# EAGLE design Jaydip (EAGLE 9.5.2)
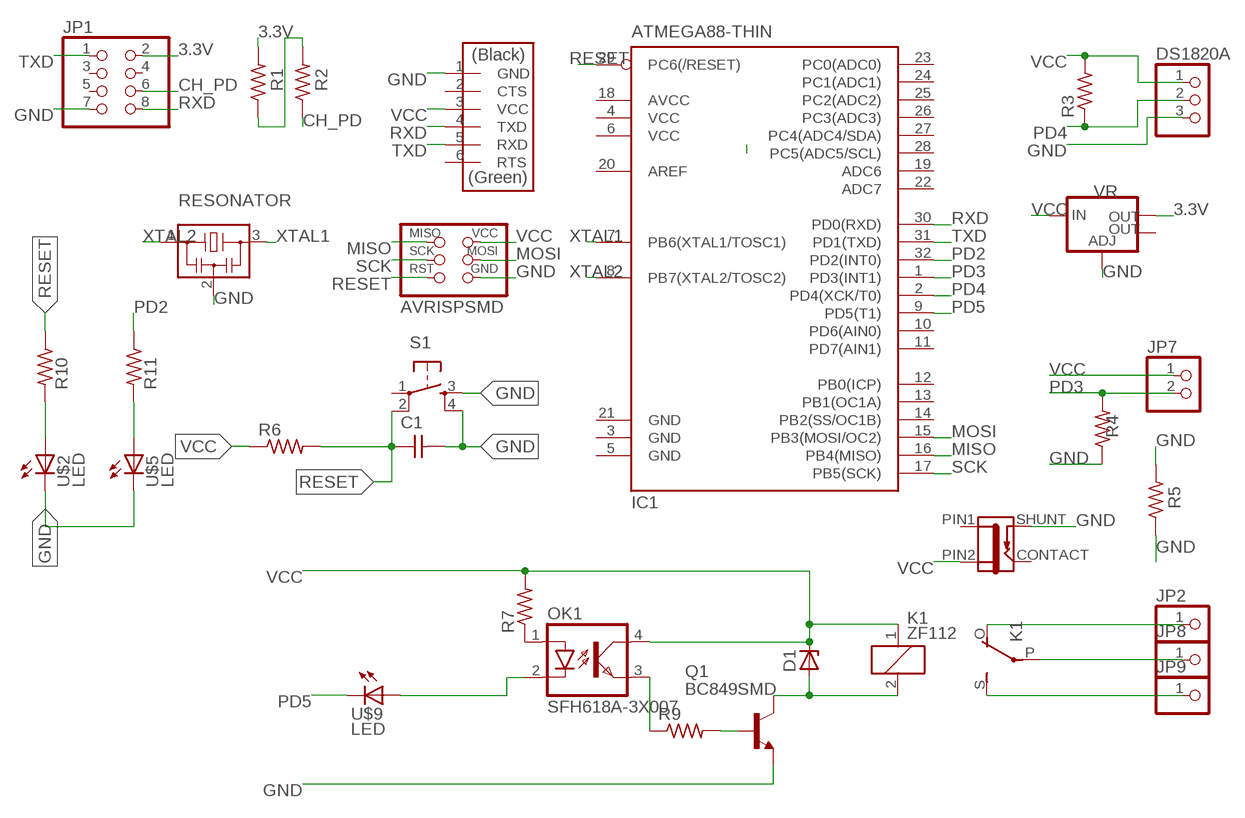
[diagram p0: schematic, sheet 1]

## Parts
C1  CAP-UNPOLARIZED  [C1206]
D1  ZENER_DIODESOD123  [SOD123]
DS1820A  PINHD-1X3  [1X03]
IC1  ATMEGA88-THIN  [TQFP32-08THIN]
J1  JACK-2.1MM  [PJ-002AH-SMT]
JP1  PINHD-2X04_2.54-SMD  [2X04SMD]
JP2  PINHD-1X01_2.00  [1X01M]
JP7  PINHD-1X02_2.54  [1X02]
JP8  PINHD-1X01_2.00  [1X01M]
JP9  PINHD-1X01_2.00  [1X01M]
K1  ZF112  [ZF112]
OK1  SFH618A-3X007  [SMD4-7]
Q1  BC849SMD  [SOT23-BEC]
R1  RES-US1206FAB  [R1206FAB]
R2  RES-US1206FAB  [R1206FAB]
R3  RES-US1206FAB  [R1206FAB]
R4  RES-US1206FAB  [R1206FAB]
R5  RES-US1206FAB  [R1206FAB]
R6  RES-US1206  [R1206]
R7  RES-US1206  [R1206]
R9  RES-US1206  [R1206]
R10  RES-US1206  [R1206]
R11  RES-US1206  [R1206]
S1  6MM_SWITCH6MM_SWITCH  [6MM_SWITCH]
U$1  AVRISPSMD  [2X03SMD]
U$2  LED  [LED1206]
U$3  RESONATOR  [EFOBM]
U$5  LED  [LED1206]
U$7  FTDI-SMD-HEADER  [1X06SMD]
U$9  LED  [LED1206]
VR  V_REG_LM1117SOT223  [SOT223]

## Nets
3.3V: JP1.2 R1.2 VR.2(OUT)
CH_PD: JP1.6 R2.1
GND: C1.2 DS1820A.3 J1.SHUNT JP1.7 Q1.E R4.1 R5.1 R5.2 S1.3(S) S1.4(S1) U$1.6(GND) U$2.2(C) U$3.2 U$5.2(C) U$7.1(GND) VR.1(ADJ)
MISO: IC1.16(PB4(MISO)) U$1.1(MISO)
MOSI: IC1.15(PB3(MOSI/OC2)) U$1.4(MOSI)
N$1: OK1.3(EMIT) R9.1
N$3: Q1.B R9.2
N$4: D1.ANODE K1.2 Q1.C
N$5: R1.1 R2.2
N$6: OK1.1(A) R7.1
N$8: OK1.2(C) U$9.1(A)
N$9: JP2.1 K1.O(2:O)
N$11: JP8.1 K1.P(2:P)
N$12: JP9.1 K1.S(2:S)
N$20: R10.2 U$2.1(A)
N$23: R11.2 U$5.1(A)
PD2: IC1.32(PD2(INT0)) R11.1
PD3: IC1.1(PD3(INT1)) JP7.2 R4.2
PD4: DS1820A.2 IC1.2(PD4(XCK/T0)) R3.1
PD5: IC1.9(PD5(T1)) U$9.2(C)
RESET: C1.1 IC1.29(PC6(/RESET)) R6.2 R10.1 S1.2(P1) U$1.5(RST)
RXD: IC1.30(PD0(RXD)) JP1.8 U$7.4(TXD)
SCK: IC1.17(PB5(SCK)) U$1.3(SCK)
TXD: IC1.31(PD1(TXD)) JP1.1 U$7.5(RXD)
VCC: D1.CATHODE DS1820A.1 J1.PIN2 JP7.1 K1.1 OK1.4(COL) R3.2 R6.1 R7.2 U$1.2(VCC) U$7.3(VCC) VR.3(IN)
XTAL1: IC1.7(PB6(XTAL1/TOSC1)) U$3.3
XTAL2: IC1.8(PB7(XTAL2/TOSC2)) U$3.1
Unconnected: IC1.10(PD6(AIN0)) IC1.11(PD7(AIN1)) IC1.12(PB0(ICP)) IC1.13(PB1(OC1A)) IC1.14(PB2(SS/OC1B)) IC1.19(ADC6) IC1.20(AREF) IC1.22(ADC7) IC1.23(PC0(ADC0)) IC1.24(PC1(ADC1)) IC1.25(PC2(ADC2)) IC1.26(PC3(ADC3)) IC1.27(PC4(ADC4/SDA)) IC1.28(PC5(ADC5/SCL)) JP1.3 JP1.4 JP1.5 S1.1(P) U$7.2(CTS) U$7.6(RTS) VR.4(OUT)

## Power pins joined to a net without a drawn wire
AVCC: IC1.18(AVCC)
CONTACT: J1.CONTACT
GND: IC1.3(GND) IC1.5(GND) IC1.21(GND)
PIN1: J1.PIN1
VCC: IC1.4(VCC) IC1.6(VCC)

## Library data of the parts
C1 = eagle_fab:CAP-UNPOLARIZED
D1 = eagle_fab:ZENER_DIODE: zener diode
DS1820A = pinhead:PINHD-1X3: PIN HEADER
IC1 = fab:ATMEGA88-THIN
J1 = fab:JACK-2.1MM: SMD DC power jack PJ-002AH-SMT As found in the fablab inventory. Made by Zaerc.
JP1 = pinhead-2:PINHD-2X04: PIN HEADER
JP2 JP8 JP9 = pinhead-2:PINHD-1X01: PIN HEADER
JP7 = pinhead-2:PINHD-1X02: PIN HEADER
K1 = relay:ZF112: RELAY 1 x switch; OC_FARNELL: unknown; OC_NEWARK: unknown
OK1 = optocoupler:SFH618?*: Optocoupler, Phototransistor Output, Low Input Current Source: Data sheet; OC_FARNELL: unknown; OC_NEWARK: unknown
Q1 = transistor-npn:BC849*: NPN Transistor
R1-R5 = fab:RES-US: Resistor (US Symbol)
R6 R7 R9-R11 = eagle_fab:RES-US: Resistor (US Symbol)
S1 = eagle_fab:6MM_SWITCH: OMRON SWITCH
U$1 = fab:AVRISP
U$2 U$5 U$9 = eagle_fab:LED: LED
U$3 = fab:RESONATOR
U$7 = eagle_fab:FTDI-SMD-HEADER
VR = fab:V_REG_LM1117: Voltage Regulator LM1117 Standard adjustable voltage regulator but in SMD form. Spark Fun Electronics SKU : COM-00595; PROD_ID: VREG-08170

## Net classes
0 default: width 0.152 mm, clearance 0.4 mm

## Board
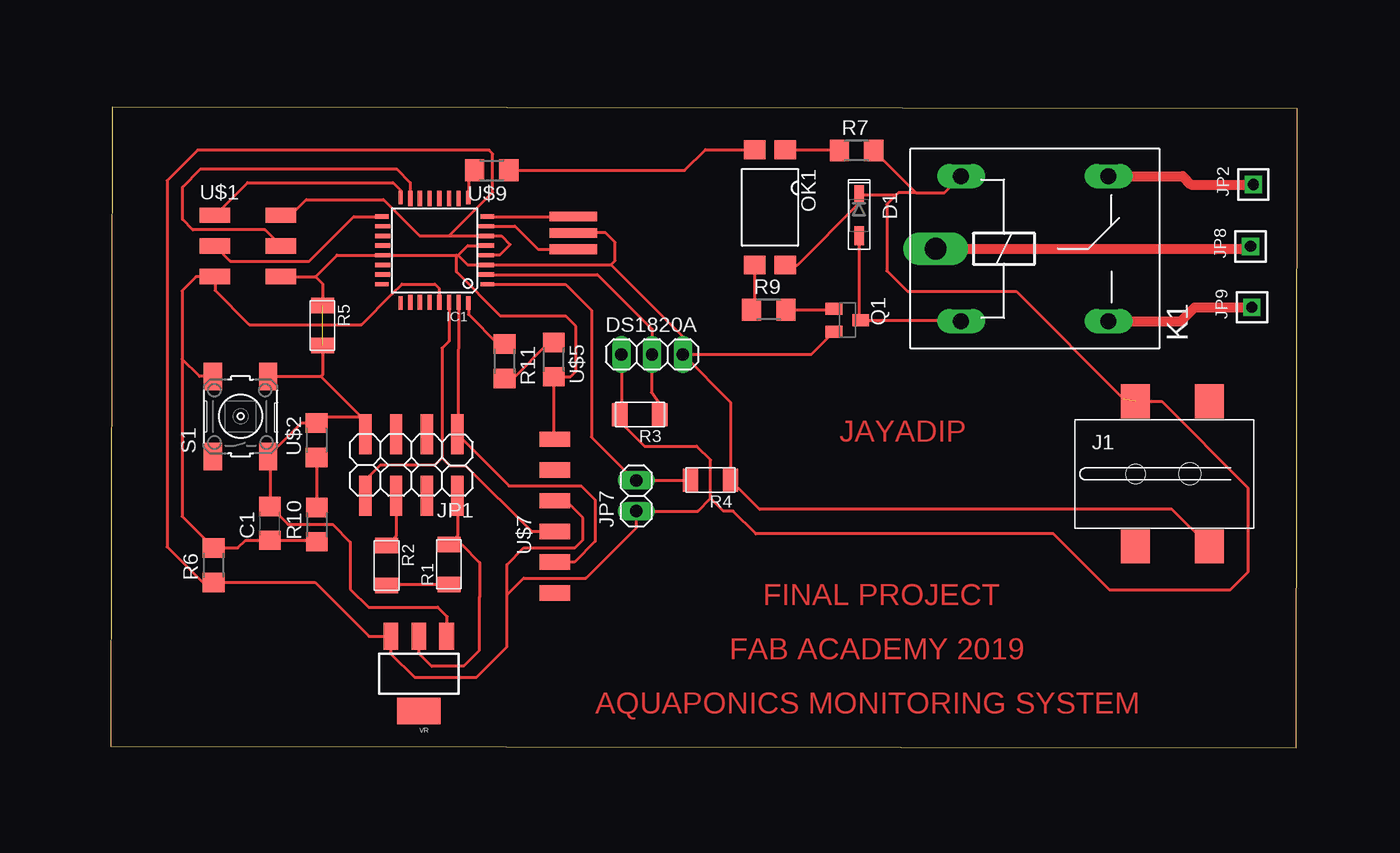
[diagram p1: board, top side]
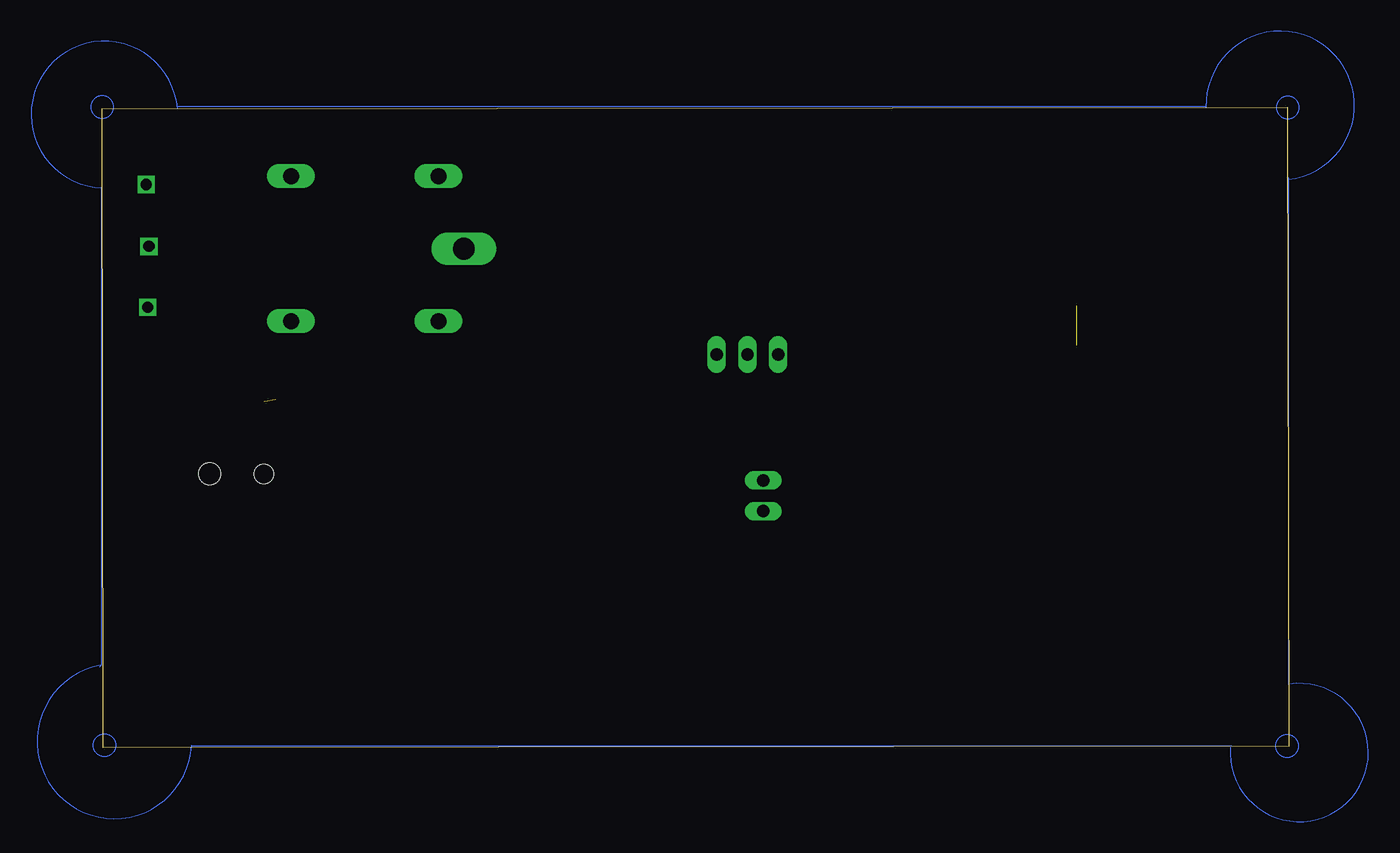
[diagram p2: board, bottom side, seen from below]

Size 98.16 x 52.96 mm. Coordinates in mm from the lower left corner, seen from the top.
Outline: 0,0.13 98.07,0 98.16,52.83 0.09,52.96 0,0.13
Copper layers (1*16): Top 0.035mm / dielectric 1.5mm / Bottom 0.035mm
Design rules "default": minimum track width 6mil, minimum drill 0.35mm, track to track 6mil, track to pad 6mil, pad to pad 6mil, via to via 6mil, smd to smd 6mil, copper to edge 40mil, drill to drill 6mil, minimum pad ring 10mil, minimum via ring 8mil, stop-mask expansion 4mil, vias tented up to drill 0mil, thermal gap 10mil

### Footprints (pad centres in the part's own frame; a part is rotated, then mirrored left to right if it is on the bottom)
C1206 = smd 1.6 x 1.8: 1 -1.4,0; 2 1.4,0
SOD123 = smd 1.6 x 0.8: ANODE 1.7,0; CATHODE -1.7,0
1X03 = drill 1.016 long: 1 -2.54,0; 2 0,0; 3 2.54,0
TQFP32-08THIN = smd 1.118 x 0.356: 1 -4.369,2.8; 8 -4.369,-2.8; 17 4.369,-2.8; 24 4.369,2.8 | smd 1.27 x 0.356: 2 -4.293,2; 3 -4.293,1.2; 4 -4.293,0.4; 5 -4.293,-0.4; 6 -4.293,-1.2; 7 -4.293,-2; 18 4.293,-2; 19 4.293,-1.2; 20 4.293,-0.4; 21 4.293,0.4; 22 4.293,1.2; 23 4.293,2 | smd 0.356 x 1.118: 9 -2.8,-4.369; 16 2.8,-4.369; 25 2.8,4.369; 32 -2.8,4.369 | smd 0.356 x 1.27: 10 -2,-4.293; 14 1.2,-4.293; 15 2,-4.293; 26 2,4.293; 27 1.2,4.293; 31 -2,4.293 | smd 0.35 x 1.27: 11 -1.2,-4.293; 12 -0.4,-4.293; 13 0.4,-4.293; 28 0.4,4.293; 29 -0.4,4.293; 30 -1.2,4.293
PJ-002AH-SMT = smd 2.4 x 2.8: CONTACT -2.4,-6; PIN1 3.7,6; PIN2 -2.4,6; SHUNT 3.7,-6 | hole 1.6: -2.4,0 | hole 1.8: 2.1,0
2X04SMD = smd 1.016 x 3.302: 1 -1.27,-3.81; 2 -1.27,1.27; 3 1.27,-3.81; 4 1.27,1.27; 5 3.81,-3.81; 6 3.81,1.27; 7 6.35,-3.81; 8 6.35,1.27
1X01M = drill 0.914 square: 1 0,0
1X02 = drill 1.016 long: 1 -1.27,0; 2 1.27,0
ZF112 = drill 1.321 long: 1 -6.096,5.994; 2 -6.096,-5.994; O 6.096,5.994; S 6.096,-5.994 | drill 1.803 long: P -8.204,0
SMD4-7 = smd 1.78 x 1.55: 1 -1.27,-4.77; 2 1.27,-4.77; 3 1.27,4.77; 4 -1.27,4.77
SOT23-BEC = smd 1 x 1.4: B -0.95,-1.1; C 0,1.1; E 0.95,-1.1
R1206FAB = smd 1.27 x 1.905: 1 -1.651,0; 2 1.651,0
R1206 = smd 1.6 x 1.803: 1 -1.422,0; 2 1.422,0
6MM_SWITCH = smd 2.286 x 1.524: 1 -3.302,2.286; 2 3.302,2.286; 3 -3.302,-2.286; 4 3.302,-2.286
2X03SMD = smd 2.54 x 1.27: 1 -2.54,2.54; 2 2.92,2.54; 3 -2.54,0; 4 2.92,0; 5 -2.54,-2.54; 6 2.92,-2.54
LED1206 = smd 1.6 x 1.803: 1 -1.422,0; 2 1.422,0
EFOBM = smd 0.8 x 3.9: 1 -1.35,0; 2 0,0; 3 1.35,0
1X06SMD = smd 2.54 x 1.27: 1 0,6.35; 2 0,3.81; 3 0,1.27; 4 0,-1.27; 5 0,-3.81; 6 0,-6.35
SOT223 = smd 1.219 x 2.235: 1 -2.311,-3.099; 2 0,-3.099; 3 2.311,-3.099 | smd 3.6 x 2.2: 4 0,3.099

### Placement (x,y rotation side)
C1  13.15,18.54 90 top
D1  61.89,44.03 270 top
DS1820A  44.77,32.52 0 top
IC1  26.77,41.12 180 top
J1  87.16,22.63 0 top
JP1  27.4,22.1 180 top
JP2  94.52,46.57 0 top
JP7  43.46,20.83 90 top
JP8  94.28,41.45 0 top
JP9  94.4,36.42 0 top
K1  76.43,41.26 0 top
OK1  54.52,44.67 180 top
Q1  60.93,35.36 270 top
R1  27.97,15.15 90 top
R2  22.81,15.05 270 top
R3  43.76,27.53 180 top
R4  49.6,22.12 180 top
R5  17.5,34.91 270 top
R6  8.49,15.09 90 top
R7  61.69,49.37 0 top
R9  54.42,36.22 0 top
R10  17.04,18.44 90 top
R11  32.58,31.95 270 top
S1  10.72,27.39 90 top
U$1  11.15,41.49 0 top
U$2  17.02,25.42 90 top
U$3  38.25,42.57 270 top
U$5  36.63,32.09 270 top
U$7  36.71,19.14 0 top
U$9  31.51,47.74 180 top
VR  25.47,6.11 180 top

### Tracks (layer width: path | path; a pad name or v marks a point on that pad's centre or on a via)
3.3V
  Top 0.254: JP1.2 28.67,17.5 R1.2 29.01,16.8 30.51,15.3 30.51,12.46 30.5,12.45 30.5,8.04 29.22,6.76 26.61,6.76 26.55,6.7 25.47,7.79 VR.2
CH_PD
  Top 0.254: JP1.6 23.59,17.49 R2.1
GND  (1 unrouted)
  Top 0.152: IC1.21 22.5,40.74
  Top 0.254: 16.93,38.95 18.7,40.72 IC1.21 28.58,40.72 | 17.36,30.69 S1.4 13.01,31.4 12.93,31.48 | JP1.7 21.05,27.01 20.7,27.35 | 17.36,30.69 20.7,27.35 | 20.7,27.35 17.53,27.35 U$2.2 15.77,26.84 S1.3 13.15,23.94 C1.2 14.65,18.45 18.35,18.45 19.8,17 19.8,13.11 21.31,11.61 27.04,11.61 27.82,10.83 27.78,10.8 VR.1 | U$7.1 36.63,25.57 U$5.2 38.03,30.67 38.48,31.12 38.48,34.84 37.63,35.68 32.23,35.68 28.58,39.33 28.58,40.72 | 28.58,40.72 28.72,40.72 | IC1.5 29.52,41.52 28.72,40.72 | 28.72,40.72 29.52,39.92 IC1.3 41.36,39.92 | U$3.2 40.92,42.57 41.71,41.78 41.71,40.27 41.36,39.92 | 41.36,39.92 47.31,33.97 DS1820A.3 | DS1820A.3 51.25,28.58 R4.1 53.66,19.71 87.78,19.71 J1.SHUNT | DS1820A.3 57.94,32.52 Q1.E | U$1.6 16.93,38.95 | 16.93,38.95 17.5,38.37 R5.1 | R5.2 17.5,30.83 17.36,30.69
MISO
  Top 0.254: U$1.1 11.3,46.71 23.33,46.71 23.97,46.07 IC1.16
MOSI
  Top 0.254: U$1.4 12.74,42.82 6.78,42.82 5.92,43.68 5.92,46.36 7.41,47.85 23.65,47.85 24.77,46.73 IC1.15
N$1
  Top 0.254: OK1.3 53.25,36.48 R9.1
N$2
  Bottom 0.076: 0.02,47 arc-265 6.84,52.94
N$3
  Top 0.254: R9.2 59.74,36.22 Q1.B
N$4
  Top 0.254: D1.ANODE 61.89,35.49 Q1.C 70.24,35.36 K1.2
N$5
  Top 0.254: R2.2 22.9,13.5 R1.1
N$6
  Top 0.254: OK1.1 60.2,49.44 R7.1
N$8
  Top 0.254: U$9.1 47.47,47.74 49.18,49.44 OK1.2
N$9
  Top 0.813: K1.O 88.66,47.25 89.35,46.57 JP2.1
N$10
  Bottom 0.076: 91.92,52.82 arc-264 98.13,46.29
N$11
  Top 0.813: K1.P 94.09,41.26 JP8.1
N$12
  Top 0.813: K1.S 88.51,35.27 89.66,36.42 JP9.1
N$13
  Bottom 0.076: 98.33,6.79 arc-256 90.76,0.18
N$14
  Bottom 0.076: 4.81,0.03 arc-283 -0.06,5.25
N$15
  Bottom 0.076: 6.85,52.99 91.91,52.99 91.94,53.02
N$16
  Bottom 0.076: 98.23,46.36 98.23,6.82 98.4,6.65
N$17
  Bottom 0.076: 90.76,0.13 4.75,0.13 4.73,0.12
N$18
  Bottom 0.076: -0.02,5.21 -0.02,47.08 0.04,47.14
N$20
  Top 0.254: U$2.1 17.02,19.89 R10.2
N$23
  Top 0.254: R11.2 33.27,30.52 36.26,33.52 U$5.1
PD2
  Top 0.254: 32.58,33.74 R11.1 32.03,33.37 29.57,35.83 IC1.32
PD3
  Top 0.254: IC1.1 37.6,38.32 39.75,36.17 39.75,25.68 43.33,22.1 JP7.2 47.93,22.1 R4.2
PD4
  Top 0.254: IC1.2 40.26,39.12 44.77,34.61 DS1820A.2 44.72,32.52 44.72,29.38 45.41,28.36 R3.1
PD5
  Top 0.254: U$9.2 29.57,47.22 IC1.9
RESET
  Top 0.254: 5.88,32.13 5.88,37.78 7.05,38.95 U$1.5 8.61,37.81 11.44,34.99 20.73,34.99 23.26,37.52 23.26,37.53 24.08,38.34 26.81,38.34 27.17,37.98 IC1.29 | 5.88,32.13 5.88,19.12 R6.2 10.5,16.51 11.13,17.14 C1.1 16.92,17.14 R10.1 | S1.2 7.32,30.69 5.88,32.13
RXD
  Top 0.254: IC1.30 27.97,33.61 27.39,33.04 27.39,24.01 27.37,23.99 27.4,23.97 | 27.4,23.97 26.77,23.35 22.27,23.35 21.05,22.13 JP1.8 | 27.4,23.97 28.04,23.32 29.33,23.32 34.78,17.87 U$7.4
SCK
  Top 0.254: U$1.3 9.88,40.22 16.4,40.22 20.09,43.92 IC1.17
TXD
  Top 0.254: IC1.31 28.77,32.99 28.72,32.94 28.72,25.96 JP1.1 32.93,21.64 38.91,21.64 40.06,20.49 40.06,17.06 38.34,15.33 U$7.5
VCC  (1 unrouted)
  Top 0.254: U$1.2 14.88,44.03 16.17,45.32 22.55,45.32 25.56,42.32 27.96,42.32 | 27.96,42.32 IC1.6 32.31,42.32 33.03,41.6 32.15,40.72 IC1.4 | U$7.3 37.64,20.41 39.05,19 39.05,17.18 38.39,16.52 34.16,16.52 32.76,15.13 32.76,12.63 | 32.76,12.63 32.76,8.32 30.24,5.8 25.13,5.8 23.15,7.78 VR.3 21.34,9.21 16.89,13.67 R6.1 7.91,13.67 7.75,13.5 4.65,16.6 4.65,46.89 7.16,49.4 31.3,49.4 31.59,49.11 31.59,45.91 31.56,45.91 27.96,42.32 | DS1820A.1 42.23,27.65 R3.2 42.58,27.06 42.58,26.48 44.13,24.93 48.46,24.93 49.6,23.78 49.6,20.61 | 32.76,12.63 34.15,14.02 39.3,14.02 43.46,18.18 JP7.1 48.55,19.56 49.6,20.61 | OK1.4 56.79,39.9 61.89,45 D1.CATHODE 64.99,45.73 | 64.99,45.73 65.13,45.87 66.62,45.87 | K1.1 68.95,45.87 66.62,45.87 | R7.2 66.62,45.87 | 49.6,20.61 50.67,19.55 51.48,19.55 53.36,17.67 77.98,17.67 82.63,13.01 92.58,13.01 94.05,14.48 94.05,21.51 86.93,28.63 J1.PIN2 | 64.99,45.73 64.2,44.93 64.2,39.42 65.9,37.72 74.9,37.72 83.81,28.81
XTAL1
  Top 0.254: IC1.7 33.42,43.12 35.32,41.22 U$3.3
XTAL2
  Top 0.254: IC1.8 U$3.1
(copper drawn outside any net)
  shapes: Bottom circle x4

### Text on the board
Top: JAYADIP | FINAL PROJECT | FAB ACADEMY 2019 | AQUAPONICS MONITORING SYSTEM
